FUNCTION "Zeitschaltuhr" : VOID
TITLE = Zeitschaltuhr "Stunde / Minute"
//KNOW_HOW_PROTECT
//
//In den Lokaldatenbereich 0.0 bis 7.9 wir mit dem SFC 1 Datum und Uhrzeit aus
//der
//CPU geschrieben.
//
//BYTE 0 Jahr    Jahr
//BYTE 1 Monat   Monat
//BYTE 2 Tag     Tag
//BYTE 3 Stunde  Stunde
//BYTE 4 Minute  Minute
//BYTE 5 Sekunde Sekunde
//BYTE 6 MS1     Die zwei höherwertigen Stellen von ms
//BYTE 7 MS2_WT  Niederwertigste Stelle von ms | Wochentag =1 So.
//
//Im LW 3 Std/Min. in BCD
//
AUTHOR : 'Kleißler'
VERSION : 0.1


VAR_INPUT
  EIN_STD : INT ;
  EIN_MIN : INT ;
  AUS_STD : INT ;
  AUS_MIN : INT ;
END_VAR
VAR_OUTPUT
  Ausgang : BOOL ;
END_VAR
VAR_TEMP
  CPU_Time : DATE_AND_TIME ;    //Gelesene CPU Uhr
  error : INT ;
  Ein_Stunde : BYTE ;
  Ein_Minute : BYTE ;
  Aus_Stunde : BYTE ;
  Aus_Minute : BYTE ;
END_VAR
BEGIN
NETWORK
TITLE =

      L     #EIN_STD; // "Ein" Stunde als Int
      ITB   ; // Ganzzahl (16 Bit) wandeln in BCD
      T     #Ein_Stunde; // in Temp. eintragen als B#16#xx

      L     #EIN_MIN; // "Ein" Minute als Int
      ITB   ; // Ganzzahl (16 Bit) wandeln in BCD
      T     #Ein_Minute; // in Temp. eintragen als B#16#xx
//------------------------------------------------------------------------------------
      L     #AUS_STD; // "Aus" Stunde als Int
      ITB   ; // Ganzzahl (16 Bit) wandeln in BCD
      T     #Aus_Stunde; // in Temp. eintragen als B#16#xx

      L     #AUS_MIN; // "Aus" Minute als Int
      ITB   ; // Ganzzahl (16 Bit) wandeln in BCD
      T     #Aus_Minute; // in Temp. eintragen als B#16#xx
//------------------------------------------------------------------------------------

      CALL SFC    1 (// Lesen System-Datum und Uhrzeit
           RET_VAL                  := #error,
           CDT                      := #CPU_Time);

      L     #error; // Fehler beim lesen der Zeit ?
      L     0; // Ist der Inhalt von #error ="0"
      <>I   ; // dann ist alles OK.
      BEB   ; // BE wenn fehler beim lesen

      L     LW     3; // Stunde:Minute
      L     LW    12; // Ausschaltzeit Stunde:Minute
      <I    ;
      U(    ;
      TAK   ; // Tausche Inhalt von AKKU 1 mit AKKU 2
      L     LW    10; // Einschaltzeit Stunde:Minute
      >=I   ;
      )     ;
      SPB   set; // =1, Sprung zu "set"
//- rückseten -------------------------------------------------------
      SET   ; // VKE auf 1 setzen
      R     #Ausgang; // rücksetzen
      SPA   end;
//- Aktiv setzen ----------------------------------------------------
set:  SET   ; // VKE auf 1 setzen
      S     #Ausgang; // Ausgang ist =
end:  NOP   0;

END_FUNCTION

